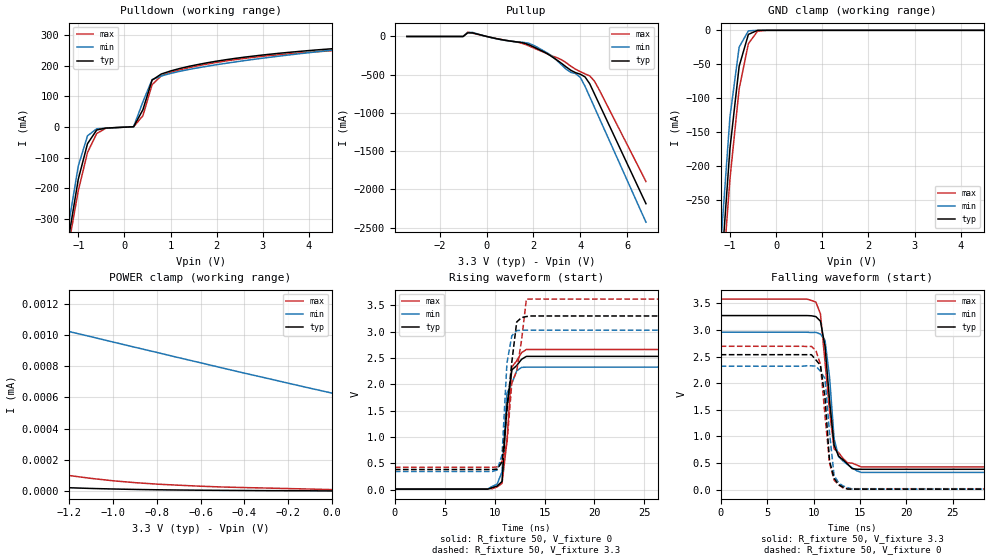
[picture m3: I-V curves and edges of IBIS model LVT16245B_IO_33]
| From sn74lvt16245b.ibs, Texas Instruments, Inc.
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|  Model LVT16245B IO_33
[Model]   LVT16245B_IO_33
Model_type  I/O
Polarity   Non-Inverting
Enable   Active-Low
Vinl = 0.8V
Vinh = 2.0V
Vmeas = 1.5V
Cref = 50pF
Rref = 500
Vref = 0
| variable   typ   min   max
C_comp   10p   NA   NA
[Temperature Range]   40   -25   100
| Ambient Temperature   25   -40   85
[Voltage range]   3.3   3.0   3.6
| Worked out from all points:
|   slope of the pulldown table from 0 to 0.495 V, typ, clamps not added: 4.82 ohm
|   slope of the pullup table from 0 to 0.495 V, typ, clamps not added: 14.8 ohm
|   GND clamp passes 1 mA (typ) near -0.43 V on its own axis
|   rising waveform, R_fixture 50, V_fixture 0: 20-80 % time 682ps typ, 530ps min, 650ps max; typ from 0.013 V to 2.53 V
|   falling waveform, R_fixture 50, V_fixture 3.3: 20-80 % time 906ps typ, 867ps min, 1.08ns max; typ from 3.27 V to 0.384 V
|   rising waveform, R_fixture 50, V_fixture 3.3: 20-80 % time 946ps typ, 513ps min, 1.47ns max; typ from 0.386 V to 3.3 V
|   falling waveform, R_fixture 50, V_fixture 0: 20-80 % time 765ps typ, 743ps min, 853ps max; typ from 2.54 V to 0.01 V
[Pullup]
|   Voltage   I(typ)   I(min)   I(max)
-3.4V     90.1uA     78.94uA    135.2uA
-1V       79.62uA    71.59uA    86.94uA
-800mV    47.49mA    51.1mA     57.38mA
1.8V      -107.5mA   -89.33mA   -122.5mA
2.6V      -226.3mA   -216.2mA   -230.6mA
3.2V      -352mA     -371.1mA   -304.9mA
3.6V      -443.1mA   -470.2mA   -389.9mA
3.8V      -473.8mA   -485.5mA   -428.6mA
4V        -493.9mA   -534.8mA   -461.1mA
4.2V      -529mA     -651mA     -488.8mA
4.6V      -748.7mA   -924.8mA   -582.9mA
6.8V      -2.188A    -2.43A     -1.898A
[Pulldown]
|   Voltage   I(typ)   I(min)   I(max)
-3.4V     -2.721A    -2.943A    -2.518A
-1.2V     -352.5mA   -309.7mA   -377.4mA
-1V       -170.2mA   -126.8mA   -207.5mA
-800mV    -54.04mA   -28.31mA   -82.76mA
-600mV    -9.301mA   -5.339mA   -20.73mA
-400mV    -3.022mA   -3.332mA   -3.596mA
200mV     1.397mA    1.529mA    1.373mA
400mV     56.53mA    82.29mA    37.09mA
600mV     153.4mA    154.9mA    138.4mA
800mV     173.2mA    166.8mA    167.5mA
2.6V      228.1mA    216.8mA    224.1mA
6.8V      295.3mA    332.9mA    278.4mA
[GND Clamp]
|   Voltage   I(typ)   I(min)   I(max)
-3.4V     -2.846A    -3.074A    -2.676A
-1.2V     -364.6mA   -317.6mA   -400.6mA
-1V       -174.1mA   -127.6mA   -219mA
-800mV    -52.87mA   -24.58mA   -85.92mA
-600mV    -5.932mA   -770.2uA   -19.62mA
-400mV    -32.68uA   -724.4nA   -1.146mA
-200mV    -27.08nA   -321.4nA   -4.839uA
5V        69.45nA    1.303uA    153.6nA
[POWER Clamp]
|   Voltage   I(typ)   I(min)   I(max)
-3.4V     510.6uA    7.026uA    1.589mA
-2.8V     1.593uA    1.817uA    17.48uA
-2.7V     1.092uA    1.708uA    8.039uA
-2.6V     778.5nA    1.623uA    4.905uA
-2.5V     568.1nA    1.551uA    3.26uA
-2.2V     243.1nA    1.39uA     1.192uA
-2.1V     187nA      1.346uA    888.4nA
-2V       145nA      1.303uA    669.7nA
-1.7V     69.45nA    1.187uA    310.4nA
-1.4V     33.36nA    1.092uA    153.6nA
-900mV    9.697nA    922.3nA    53.29nA
0V        102.7pA    627.7nA    8.466nA
[ramp]
| variable   typ   min   max
dV/dt_r   1.356E+00/8.200E-10  1.266E+00/7.800E-10  1.452E+00/8.400E-10
dV/dt_f   1.710E+00/6.100E-10  1.566E+00/4.900E-10  1.824E+00/6.800E-10
R_load = 50
[Rising Waveform]
R_fixture = 50
V_fixture = 0
V_fixture_min = 0
V_fixture_max = 0
C_fixture = 0
L_fixture = 0
|   Time   V(typ)   V(min)   V(max)
0s        12.64mV    12.94mV    20.38mV
9.277ns   12.64mV    12.94mV    20.38mV
10.25ns   71.66mV    108mV      55.58mV
10.74ns   158.2mV    344.5mV    122.8mV
11.23ns   1.583V     1.834V     917.5mV
11.72ns   2.276V     2.021V     2.33V
12.21ns   2.359V     2.26V      2.449V
12.7ns    2.478V     2.324V     2.604V
13.18ns   2.533V     2.329V     2.664V
49.71ns   2.533V     2.329V     2.664V
[Falling Waveform]
R_fixture = 50
V_fixture = 3.3
V_fixture_min = 3
V_fixture_max = 3.6
C_fixture = 0pf
L_fixture = 0nH
|   Time   V(typ)   V(min)   V(max)
0s        3.272V     2.959V     3.582V
10.25ns   3.252V     2.956V     3.525V
10.74ns   3.166V     2.925V     3.303V
11.23ns   2.696V     2.808V     2.403V
11.72ns   1.674V     2.115V     1.478V
12.21ns   837.1mV    957.4mV    766.5mV
12.7ns    627.9mV    620.3mV    696.3mV
13.67ns   480.2mV    470.7mV    504.9mV
15.14ns   383.6mV    325.6mV    428.1mV
49.71ns   383.6mV    325.6mV    428.1mV
[Rising Waveform]
R_fixture = 50
V_fixture = 3.3
V_fixture_min = 3
V_fixture_max = 3.6
C_fixture = 0pf
L_fixture = 0nH
|   Time   V(typ)   V(min)   V(max)
0s        386.3mV    349.2mV    427.7mV
9.766ns   386.3mV    349.2mV    427.7mV
10.25ns   391.8mV    375.5mV    434.8mV
10.74ns   529.8mV    662.7mV    539.9mV
11.23ns   1.498V     2.403V     877.9mV
11.72ns   2.425V     2.924V     2.027V
12.21ns   3.186V     3.022V     2.259V
12.7ns    3.27V      3.03V      2.845V
13.18ns   3.289V     3.03V      3.621V
49.71ns   3.3V       3.03V      3.621V
[Falling Waveform]
R_fixture = 50
V_fixture = 0
V_fixture_min = 0
V_fixture_max = 0
C_fixture = 0pf
L_fixture = 0nH
|   Time   V(typ)   V(min)   V(max)
0s        2.537V     2.32V      2.695V
9.766ns   2.537V     2.327V     2.692V
10.25ns   2.438V     2.323V     2.617V
10.74ns   2.336V     2.225V     2.351V
11.23ns   1.726V     2.086V     1.389V
11.72ns   534.5mV    1.062V     500mV
12.21ns   214.7mV    265.5mV    178.6mV
13.18ns   45.46mV    69.1mV     31.28mV
14.16ns   10.14mV    12.09mV    18.79mV
49.71ns   10.14mV    12.09mV    18.79mV
